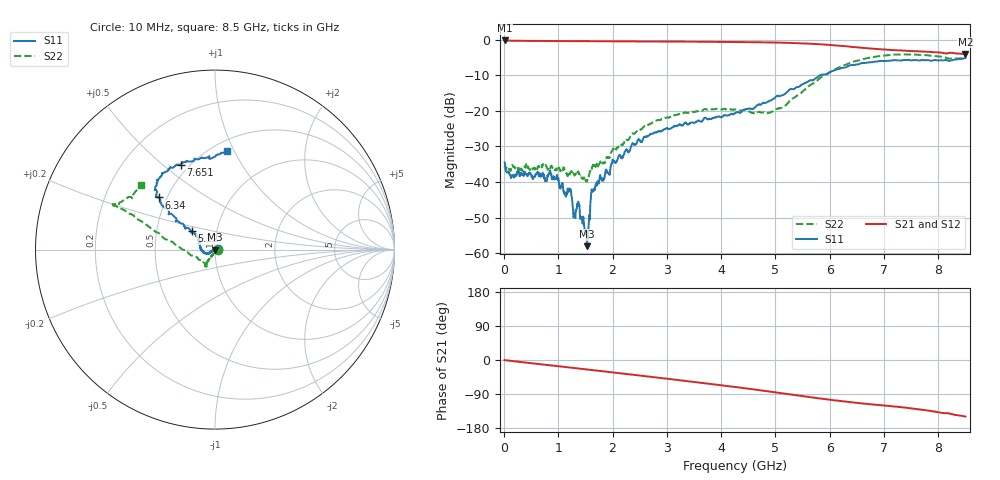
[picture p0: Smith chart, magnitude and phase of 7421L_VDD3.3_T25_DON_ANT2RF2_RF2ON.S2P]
!Agilent Technologies,E5071C,MY46417908,A.11.23
!Date: Thu Feb 25 16:17:12 2021
!Data & Calibration Information:
!Freq	S11:SOLT2(ON)	S21:SOLT2(ON)	S12:SOLT2(ON)	S22:SOLT2(ON)
!PortZ  Port1:50+j0  Port2:50+j0
!Above PortZ is port z conversion or system Z0 setting when saving the data.
!When reading, reference impedance value at option line is always used.
# Hz S dB R 50
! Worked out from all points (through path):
!   1601 points, 10 MHz to 8.5 GHz, reference 50 ohm
!   highest |S21| = -0.18 dB at 10 MHz (marker M1); lowest = -4.0 dB at 8.5 GHz (marker M2)
!   group delay of S21, straight-line fit = 48.4 ps
!   lowest |S11| = -58.0 dB at 1.528 GHz (marker M3), VSWR 1.00, Z = 49.9 - j0.0255 ohm
!   |S11| at or under -10 dB: start of sweep to 5.819 GHz
!   |S22| runs from -39.8 to -4.1 dB; largest |S21 - S12| = 0.0065
!   S11 on the Smith chart (normalised r, x): 10 MHz: 1.04, +0.00; 5.12 GHz: 0.75, +0.16; 6.34 GHz: 0.45, +0.32; 7.651 GHz: 0.45, +0.58; 8.5 GHz: 0.59, +0.94
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1e7  -34.48 2.4  -0.18 -0.4  -0.18 -0.4  -35.92 -7.5
1.532688e8  -38.18 5.9  -0.26 -2.8  -0.26 -2.8  -35.20 0.8
9.65125e8  -38.51 46.7  -0.33 -15.9  -0.34 -15.9  -36.69 12.2
1.124312e9  -42.95 54.9  -0.34 -18.4  -0.35 -18.4  -37.02 -16.1
1.209212e9  -42.25 56.1  -0.34 -19.8  -0.34 -19.8  -37.84 -3.1
1.299419e9  -48.69 54.9  -0.35 -21.3  -0.36 -21.3  -38.20 -25.4
1.363094e9  -45.80 112.0  -0.36 -22.3  -0.36 -22.3  -37.18 -31.5
1.426769e9  -49.88 135.1  -0.36 -23.3  -0.36 -23.3  -38.82 -43.8
1.527588e9  -58.03 -168.2  -0.36 -25.0  -0.36 -25.0  -39.83 -74.1
1.628406e9  -42.75 -159.5  -0.37 -26.7  -0.37 -26.7  -35.64 -80.7
1.734531e9  -40.21 -170.1  -0.38 -28.4  -0.38 -28.4  -35.48 -84.0
2.376588e9  -29.12 -146.7  -0.42 -39.0  -0.42 -39.0  -26.38 -121.2
2.843538e9  -25.77 -154.3  -0.46 -46.8  -0.46 -46.8  -22.51 -122.8
3.719069e9  -21.96 -177.8  -0.55 -61.7  -0.55 -61.8  -19.45 -122.8
4.255e9  -20.62 156.3  -0.63 -71.2  -0.63 -71.2  -19.55 -117.1
4.870525e9  -17.38 141.7  -0.73 -82.7  -0.73 -82.7  -20.61 -135.9
5.119919e9  -15.62 142.1  -0.82 -87.6  -0.81 -87.6  -19.05 -158.7
5.671769e9  -11.41 144.0  -1.13 -98.5  -1.11 -98.4  -12.42 169.9
6.340356e9  -7.39 137.2  -1.88 -110.6  -1.90 -110.7  -6.69 158.5
7.088538e9  -5.88 126.3  -2.80 -121.3  -2.79 -121.4  -4.30 156.3
7.651e9  -5.83 112.0  -3.27 -130.4  -3.29 -130.3  -4.24 156.2
8.5e9  -5.11 83.0  -4.01 -149.2  -4.04 -149.6  -5.22 138.9
